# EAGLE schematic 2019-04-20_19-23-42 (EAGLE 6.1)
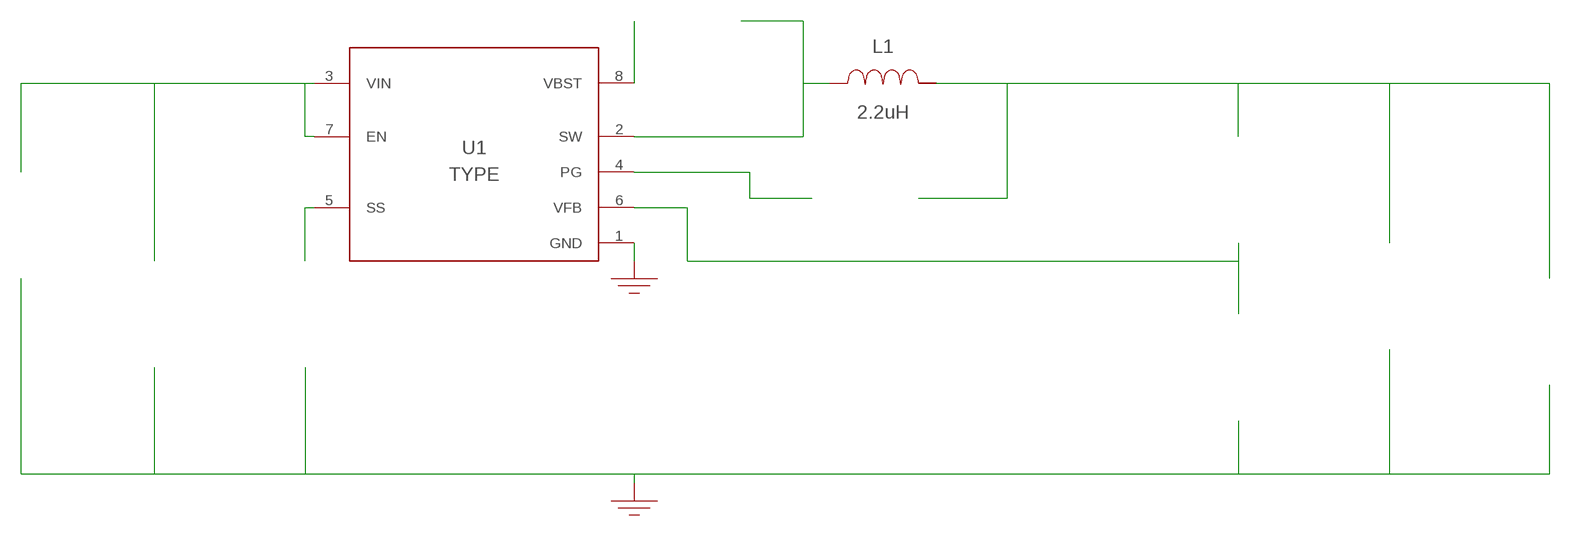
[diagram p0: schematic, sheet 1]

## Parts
CBST  100nF  C0603C104Z3VACTUC0603C104Z3VACTU  [0603]  (not placed on a sheet)
CIN  22uF  C2012X5R1V226M125ACC2012X5R1V226M125AC  [0805]  (not placed on a sheet)
COUT  47uF  C3216X5R1E476M160ACC3216X5R1E476M160AC  [1206]  (not placed on a sheet)
CSS  8.2nF  GRM033R71A822KA01DGRM033R71A822KA01D  [0201]  (not placed on a sheet)
GND  WB_GND  WB_GNDWB_GND  [WB_GND]
GND2  WB_GND  WB_GNDWB_GND  [WB_GND]
IOUT  WB_CURRENT_LOAD  WB_CURRENT_LOADWB_CURRENT_LOAD  [WB_CURRENT_LOAD]  (not placed on a sheet)
L1  2.2uH  VLP8040T-2R2NVLP8040T-2R2N  [VLP8040]
RFBB  10k  RC0201FR-0710KLRC0201FR-0710KL  [0201]  (not placed on a sheet)
RFBT  33.2k  ERJ-6ENF3322VERJ-6ENF3322V  [0805]  (not placed on a sheet)
RPG  100k  CRCW0402100KFKEDCRCW0402100KFKED  [0402]  (not placed on a sheet)
U1  TPS563210ADDFR  TPS563210ADDFRTPS563210ADDFR  [DDF0008A_N]
VIN  WB_BATTERY  WB_BATTERYWB_BATTERY  [WB_BATTERY]  (not placed on a sheet)

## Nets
0: Cin.2@2 Cout.2@2 Css.2@2 GND2.1 GND.1 Iout.-@2 Rfbb.2@2 U1.1(GND) Vin.-@2
1: Rpg.2@2 U1.4(PG)
2: Rfbb.1@1 Rfbt.2@2 U1.6(VFB)
3: Cin.1@1 U1.3(VIN) U1.7(EN) Vin.+@1
4: Cbst.1@1 L1.1 U1.2(SW)
5: Css.1@1 U1.5(SS)
6: Cout.1@1 Iout.+@1 L1.2 Rfbt.1@1 Rpg.1@1
7: Cbst.2@2 U1.8(VBST)
Unconnected: CBST.1 CBST.2 CIN.1 CIN.2 COUT.1 COUT.2 CSS.1 CSS.2 IOUT.1(+) IOUT.2(-) RFBB.1 RFBB.2 RFBT.1 RFBT.2 RPG.1 RPG.2 VIN.1(+) VIN.2(-)

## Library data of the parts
CBST = AcceleratedDesigns_Lib:C0603C104Z3VACTU; Cap: 1.0E-7; ESR: 0.0; IRMS: 0.0; Manufacturer_Name: Kemet; Manufacturer_Part_Number: C0603C104Z3VACTU; VDC: 25.0; Vendor: Kemet
CIN = AcceleratedDesigns_Lib:C2012X5R1V226M125AC; Cap: 2.2E-5; Datasheet_URL: https://product.tdk.com/en/search/capacitor/ceramic/mlcc/info?part%5Fno%3DC2012X5R1V226M125AC; ESR: 0.00205; IRMS: 4.55587; Manufacturer_Name: TDK; Manufacturer_Part_Number: C2012X5R1V226M125AC; VDC: 35.0; Vendor: TDK
COUT = AcceleratedDesigns_Lib:C3216X5R1E476M160AC; Cap_F: 0.000047; Manufacturer_Name: TDK; Manufacturer_Part_Number: C3216X5R1E476M160AC; MountType: SMT; RoHS: Y; VDC_V: 25
CSS = AcceleratedDesigns_Lib:GRM033R71A822KA01D; Cap: 8.2E-9; ESR: 0.0; IRMS: 0.0; Manufacturer_Name: MuRata; Manufacturer_Part_Number: GRM033R71A822KA01D; VDC: 10.0; Vendor: MuRata
GND GND2 = AcceleratedDesigns_Lib:WB_GND; Manufacturer_Name: WB_GND; Manufacturer_Part_Number: WB_GND; PowerPortType: POWER_GROUND; Value: Value
IOUT = AcceleratedDesigns_Lib:WB_CURRENT_LOAD; Manufacturer_Name: WB_CURRENT_LOAD; Manufacturer_Part_Number: WB_CURRENT_LOAD; PowerPortType: POWER_GROUND; Value: Value
L1 = AcceleratedDesigns_Lib:VLP8040T-2R2N; DCR: 0.015; Datasheet_URL: http://www.tdk.co.jp/tjfx01/j531_vlp.pdf; Description: Unknown; IDC: 6.7; L: 2.2E-6; Manufacturer: TDK; Manufacturer_Name: TDK; Manufacturer_Part_Number: VLP8040T-2R2N; PACKAGE_DESIGNATOR: VLP8040; Vendor: TDK
RFBB = AcceleratedDesigns_Lib:RC0201FR-0710KL; Datasheet_URL: http://www.yageo.com/documents/recent/PYu%2DRC%5FGroup%5F51%5FRoHS%5FL%5F5.pdf; Manufacturer_Name: Yageo; Manufacturer_Part_Number: RC0201FR-0710KL; Power: 0.05; Resistance: 10000.0; Tolerance: 1.0; Vendor: Yageo America
RFBT = AcceleratedDesigns_Lib:ERJ-6ENF3322V; Manufacturer_Name: Panasonic; Manufacturer_Part_Number: ERJ-6ENF3322V; Power: 0.125; Resistance: 33200.0; Tolerance: 1.0; Vendor: Panasonic
RPG = AcceleratedDesigns_Lib:CRCW0402100KFKED; Manufacturer_Name: Vishay-Dale; Manufacturer_Part_Number: CRCW0402100KFKED; Power: 0.063; Resistance: 100000.0; Tolerance: 1.0; Vendor: Vishay-Dale
U1 = AcceleratedDesigns_Lib:TPS563210ADDFR; Manufacturer: Texas Instruments; Manufacturer_Name: Texas Instruments; Manufacturer_Part_Number: TPS563210ADDFR; PartNumber: TPS563210ADDFR; RefDes: RefDes; TYPE: TYPE; Value: Value
VIN = AcceleratedDesigns_Lib:WB_BATTERY; Manufacturer_Name: WB_BATTERY; Manufacturer_Part_Number: WB_BATTERY; PowerPortType: POWER_GROUND; Value: Value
